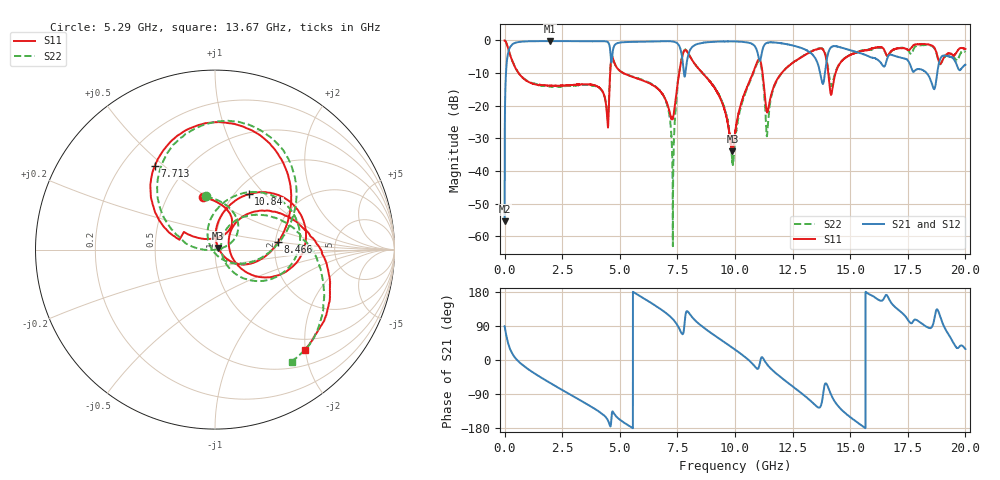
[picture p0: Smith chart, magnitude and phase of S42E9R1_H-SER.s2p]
!{S42E9R1}
!Johanson Technology Inc.
!www.johansontechnology.com
!Test Board Conditions:
!Substrate Type  RO4350B
!Substrate Thickness  50 mil
!Substrate Dk  3.66
!TL Type: GCPW
!TL Trace Width  60 mil
!TL Gap  10 mil
!Electrode orientation  Horizontal
!DUT TOPOLOGY	SERIES
!Mounting Pad LxW  14x55 mil
! Created Wed Nov 25 21:51:52 2020
# khz S ma R 50
! 2 Port Network Data from SP1.SP block
! freq  magS11  angS11  magS21  angS21  magS12  angS12  magS22  angS22
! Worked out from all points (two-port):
!   20001 points, 300 kHz to 20 GHz, reference 50 ohm
!   highest |S21| = -0.19 dB at 1.962 GHz (marker M1); lowest = -55.4 dB at 300 kHz (marker M2)
!   |S21| within 3 dB of the highest: 175.5 MHz to 4.585 GHz (4.41 GHz wide, 185 % of centre); 4.697 GHz to 7.654 GHz (2.957 GHz wide, 47.9 % of centre)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
!   lowest |S11| = -34.0 dB at 9.891 GHz (marker M3), VSWR 1.04, Z = 51.8 + j1.01 ohm
!   |S11| at or under -10 dB: 607.8 MHz to 4.581 GHz (3.973 GHz wide, 153 % of centre); 5.156 GHz to 7.577 GHz (2.421 GHz wide, 38 % of centre); 8.587 GHz to 10.78 GHz (2.19 GHz wide, 22.6 % of centre)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
!   |S22| runs from -63.0 to 0.0 dB; largest |S21 - S12| = 0.019
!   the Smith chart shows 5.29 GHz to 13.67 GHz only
!   S11 on the Smith chart (normalised r, x): 5.29 GHz: 0.75, +0.48; 7.713 GHz: 0.34, +0.47; 8.466 GHz: 2.07, +0.19; 10.84 GHz: 1.15, +0.82; 13.67 GHz: 0.78, -1.99
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300  0.9987 -0.3  0.001702 89.5  0.001737 90.6  0.9968 -0.1
105300  0.8601 -34.3  0.5046 55.5  0.5062 55.4  0.8609 -34.3
228300  0.6194 -59.7  0.7776 29.9  0.7776 29.9  0.6215 -59.7
1962300  0.2027 -150.3  0.9782 -60.1  0.9773 -60.0  0.1993 -149.9
3334300  0.2123 157.6  0.9741 -108.1  0.9729 -108.1  0.2079 165.6
4439300  0.07685 131.6  0.9613 -154.6  0.9617 -154.5  0.08291 143.2
4683300  0.5565 156.7  0.6394 -135.7  0.6392 -135.8  0.56 156.3
5290300  0.2999 102.4  0.9447 -169.4  0.9457 -169.5  0.3012 99.9
6667300  0.1791 57.9  0.9721 138.5  0.9708 138.5  0.1815 44.3
7297300  0.06364 110.4  0.9637 108.1  0.9633 108.1  0.003042 -1.2
7713300  0.5744 125.7  0.5269 68.1  0.5247 68.1  0.5866 118.3
8466300  0.354 6.6  0.9016 93.8  0.8978 93.8  0.3544 5.7
9891300  0.01992 29.5  0.9672 32.1  0.9663 32.2  0.0136 -128.7
1.00003e7  0.03781 77.0  0.9649 27.4  0.9675 27.5  0.02746 150.2
1.08423e7  0.3617 58.6  0.829 -15.5  0.8272 -15.3  0.3472 64.3
1.11113e7  0.4788 -4.6  0.5159 1.4  0.5155 1.8  0.4395 -8.9
1.14073e7  0.08014 14.3  0.9231 -12.7  0.9225 -12.6  0.04016 33.0
1.33343e7  0.6808 -19.8  0.6196 -110.7  0.6263 -110.8  0.6877 -28.6
1.36673e7  0.7509 -48.2  0.3554 -125.5  0.3577 -126.0  0.7569 -55.7
1.41843e7  0.1509 -58.0  0.7948 -93.3  0.795 -93.0  0.2015 -71.7
1.66673e7  0.6033 -116.5  0.5892 163.0  0.5778 163.3  0.6047 -129.9
2e7  0.7411 143.7  0.4272 28.7  0.4302 29.4  0.6605 126.5
